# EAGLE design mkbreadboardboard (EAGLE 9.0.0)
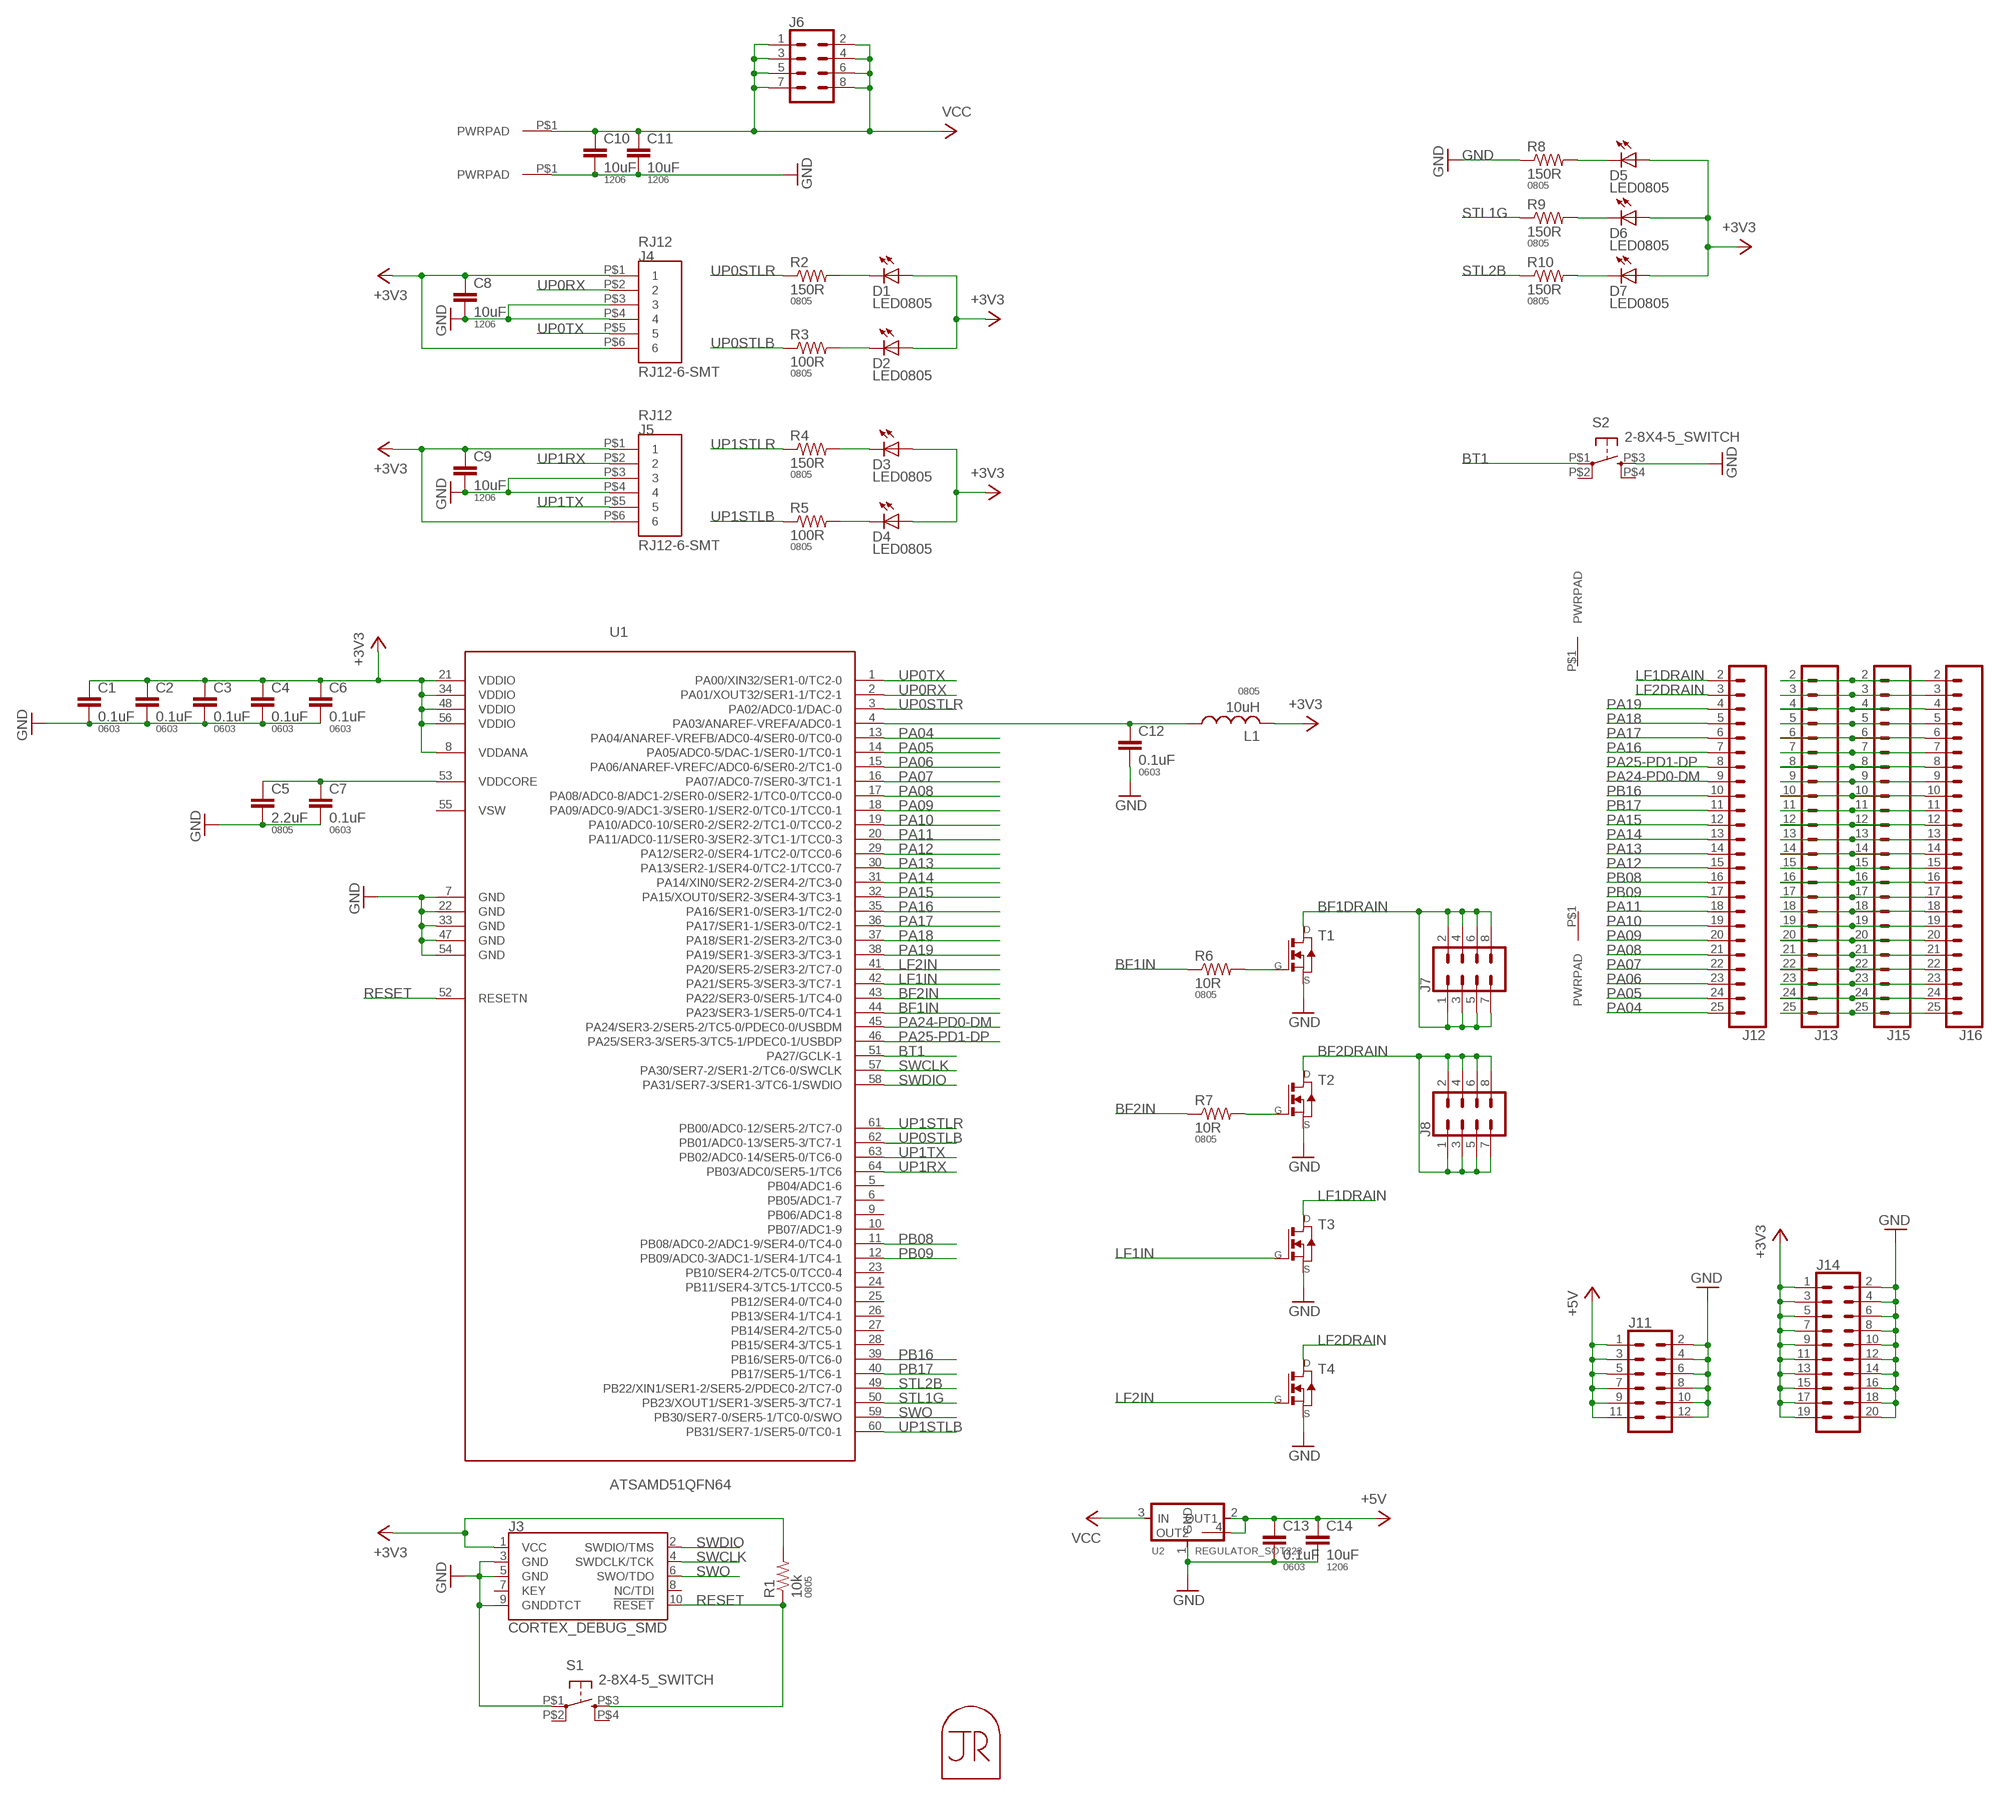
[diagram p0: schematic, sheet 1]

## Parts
C1  0.1uF  CAP0603-CAP  [0603-CAP]
C2  0.1uF  CAP0603-CAP  [0603-CAP]
C3  0.1uF  CAP0603-CAP  [0603-CAP]
C4  0.1uF  CAP0603-CAP  [0603-CAP]
C5  2.2uF  CAP0805  [0805]
C6  0.1uF  CAP0603-CAP  [0603-CAP]
C7  0.1uF  CAP0603-CAP  [0603-CAP]
C8  10uF  CAP1206  [1206]
C9  10uF  CAP1206  [1206]
C10  10uF  CAP1206  [1206]
C11  10uF  CAP1206  [1206]
C12  0.1uF  CAP0603-CAP  [0603-CAP]
C13  0.1uF  CAP0603-CAP  [0603-CAP]
C14  10uF  CAP1206  [1206]
D1  LED0805  [LED0805]
D2  LED0805  [LED0805]
D3  LED0805  [LED0805]
D4  LED0805  [LED0805]
D5  LED0805  [LED0805]
D6  LED0805  [LED0805]
D7  LED0805  [LED0805]
J1  PWRPAD  [PWRPAD_M3-PEM-MOUNT]
J2  PWRPAD  [PWRPAD_M3-PEM-MOUNT]
J3  CORTEX_DEBUG_SMD  [SAMTECH_FTSH-105-01]
J4  RJ12-6-SMT  [RJ12-6-SMT]
J5  RJ12-6-SMT  [RJ12-6-SMT]
J6  CONN_04X2  [2X4]
J7  CONN_04X2  [2X4]
J8  CONN_04X2  [2X4]
J9  PWRPADM3  [PWRPAD_3-25MM]
J10  PWRPADM3  [PWRPAD_3-25MM]
J11  CONN_06X2NO_SILK  [2X6_NOSILK]
J12  CONN_24  [1X24]
J13  CONN_24  [1X24]
J14  CONN_10X2NOSILK  [2X10_NOSILK]
J15  CONN_24  [1X24]
J16  CONN_24  [1X24]
L1  10uH  INDUCTOR-0805  [0805]
MP1  JRTOMBSTONE  [JRTOMBSTONE]
R1  10k  RESISTOR0805-RES  [0805]
R2  150R  RESISTOR0805-RES  [0805]
R3  100R  RESISTOR0805-RES  [0805]
R4  150R  RESISTOR0805-RES  [0805]
R5  100R  RESISTOR0805-RES  [0805]
R6  10R  RESISTOR0805-RES  [0805]
R7  10R  RESISTOR0805-RES  [0805]
R8  150R  RESISTOR0805-RES  [0805]
R9  150R  RESISTOR0805-RES  [0805]
R10  150R  RESISTOR0805-RES  [0805]
S1  2-8X4-5_SWITCH  [TACT-SWITCH-KMR6]
S2  2-8X4-5_SWITCH  [TACT-SWITCH-KMR6]
T1  NMOSFETTO252  [TO252]
T2  NMOSFETTO252  [TO252]
T3  NMOSFETSOT23  [SOT-23]
T4  NMOSFETSOT23  [SOT-23]
U1  ATSAMD51QFN64  [QFN-64-9X9MM]
U2  REGULATOR_SOT223  [SOT223]

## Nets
+3V3: C1.1 C2.1 C3.1 C4.1 C6.1 C8.1 C9.1 D1.1(A) D2.1(A) D3.1(A) D4.1(A) D5.1(A) D6.1(A) D7.1(A) J3.1(VCC) J4.P$1 J4.P$6 J5.P$1 J5.P$6 J14.1 J14.3 J14.5 J14.7 J14.9 J14.11 J14.13 J14.15 J14.17 J14.19 L1.2 R1.2 U1.8(VDDANA) U1.21(VDDIO) U1.34(VDDIO) U1.48(VDDIO) U1.56(VDDIO)
+5V: C13.1 C14.1 J11.1 J11.3 J11.5 J11.7 J11.9 J11.11 U2.2(OUT1) U2.4(OUT2)
BF1DRAIN: J7.1 J7.2 J7.3 J7.4 J7.5 J7.6 J7.7 J7.8 T1.3(D)
BF1IN: R6.1 U1.44(PA23/SER3-1/SER5-0/TC4-1)
BF2DRAIN: J8.1 J8.2 J8.3 J8.4 J8.5 J8.6 J8.7 J8.8 T2.3(D)
BF2IN: R7.1 U1.43(PA22/SER3-0/SER5-1/TC4-0)
BT1: S2.P$1(P) U1.51(PA27/GCLK-1)
GND: C1.2 C2.2 C3.2 C4.2 C5.2 C6.2 C7.2 C8.2 C9.2 C10.2 C11.2 C12.2 C13.2 C14.2 J2.P$1(PWRPAD) J3.3(GND) J3.5(GND) J3.9(GNDDTCT) J4.P$3 J4.P$4 J5.P$3 J5.P$4 J11.2 J11.4 J11.6 J11.8 J11.10 J11.12 J14.2 J14.4 J14.6 J14.8 J14.10 J14.12 J14.14 J14.16 J14.18 J14.20 R8.1 S1.P$1(P) S2.P$3(S) T1.2(S) T2.2(S) T3.2(S) T4.2(S) U1.7(GND) U1.22(GND) U1.33(GND) U1.47(GND) U1.54(GND) U2.1(GND)
LF1DRAIN: J12.2 T3.1(D)
LF1IN: T3.3(G) U1.42(PA21/SER5-3/SER3-3/TC7-1)
LF2DRAIN: J12.3 T4.1(D)
LF2IN: T4.3(G) U1.41(PA20/SER5-2/SER3-2/TC7-0)
N$1: J13.7 J15.7 J16.7
N$2: D1.2(C) R2.2
N$3: J13.8 J15.8 J16.8
N$4: D3.2(C) R4.2
N$5: C5.1 C7.1 U1.53(VDDCORE)
N$6: D2.2(C) R3.2
N$7: D4.2(C) R5.2
N$8: C12.1 L1.1 U1.4(PA03/ANAREF-VREFA/ADC0-1)
N$9: D5.2(C) R8.2
N$10: D6.2(C) R9.2
N$11: D7.2(C) R10.2
N$13: R6.2 T1.1(G)
N$14: R7.2 T2.1(G)
N$15: J13.2 J15.2 J16.2
N$16: J13.3 J15.3 J16.3
N$17: J13.4 J15.4 J16.4
N$18: J13.5 J15.5 J16.5
N$19: J13.6 J15.6 J16.6
N$20: J13.9 J15.9 J16.9
N$21: J13.10 J15.10 J16.10
N$22: J13.11 J15.11 J16.11
N$23: J13.12 J15.12 J16.12
N$24: J13.13 J15.13 J16.13
N$25: J13.14 J15.14 J16.14
N$26: J13.15 J15.15 J16.15
N$27: J13.16 J15.16 J16.16
N$28: J13.17 J15.17 J16.17
N$29: J13.18 J15.18 J16.18
N$30: J13.19 J15.19 J16.19
N$31: J13.20 J15.20 J16.20
N$32: J13.21 J15.21 J16.21
N$33: J13.22 J15.22 J16.22
N$34: J13.23 J15.23 J16.23
N$35: J13.24 J15.24 J16.24
N$36: J13.25 J15.25 J16.25
PA04: J12.25 U1.13(PA04/ANAREF-VREFB/ADC0-4/SER0-0/TC0-0)
PA05: J12.24 U1.14(PA05/ADC0-5/DAC-1/SER0-1/TC0-1)
PA06: J12.23 U1.15(PA06/ANAREF-VREFC/ADC0-6/SER0-2/TC1-0)
PA07: J12.22 U1.16(PA07/ADC0-7/SER0-3/TC1-1)
PA08: J12.21 U1.17(PA08/ADC0-8/ADC1-2/SER0-0/SER2-1/TC0-0/TCC0-0)
PA09: J12.20 U1.18(PA09/ADC0-9/ADC1-3/SER0-1/SER2-0/TC0-1/TCC0-1)
PA10: J12.19 U1.19(PA10/ADC0-10/SER0-2/SER2-2/TC1-0/TCC0-2)
PA11: J12.18 U1.20(PA11/ADC0-11/SER0-3/SER2-3/TC1-1/TCC0-3)
PA12: J12.15 U1.29(PA12/SER2-0/SER4-1/TC2-0/TCC0-6)
PA13: J12.14 U1.30(PA13/SER2-1/SER4-0/TC2-1/TCC0-7)
PA14: J12.13 U1.31(PA14/XIN0/SER2-2/SER4-2/TC3-0)
PA15: J12.12 U1.32(PA15/XOUT0/SER2-3/SER4-3/TC3-1)
PA16: J12.7 U1.35(PA16/SER1-0/SER3-1/TC2-0)
PA17: J12.6 U1.36(PA17/SER1-1/SER3-0/TC2-1)
PA18: J12.5 U1.37(PA18/SER1-2/SER3-2/TC3-0)
PA19: J12.4 U1.38(PA19/SER1-3/SER3-3/TC3-1)
PA24-PD0-DM: J12.9 U1.45(PA24/SER3-2/SER5-2/TC5-0/PDEC0-0/USBDM)
PA25-PD1-DP: J12.8 U1.46(PA25/SER3-3/SER5-3/TC5-1/PDEC0-1/USBDP)
PB08: J12.16 U1.11(PB08/ADC0-2/ADC1-9/SER4-0/TC4-0)
PB09: J12.17 U1.12(PB09/ADC0-3/ADC1-1/SER4-1/TC4-1)
PB16: J12.10 U1.39(PB16/SER5-0/TC6-0)
PB17: J12.11 U1.40(PB17/SER5-1/TC6-1)
RESET: J3.10(!RESET) R1.1 S1.P$3(S) U1.52(RESETN)
STL1G: R9.1 U1.50(PB23/XOUT1/SER1-3/SER5-3/TC7-1)
STL2B: R10.1 U1.49(PB22/XIN1/SER1-2/SER5-2/PDEC0-2/TC7-0)
SWCLK: J3.4(SWDCLK/TCK) U1.57(PA30/SER7-2/SER1-2/TC6-0/SWCLK)
SWDIO: J3.2(SWDIO/TMS) U1.58(PA31/SER7-3/SER1-3/TC6-1/SWDIO)
SWO: J3.6(SWO/TDO) U1.59(PB30/SER7-0/SER5-1/TC0-0/SWO)
UP0RX: J4.P$2 U1.2(PA01/XOUT32/SER1-1/TC2-1)
UP0STLB: R3.1 U1.62(PB01/ADC0-13/SER5-3/TC7-1)
UP0STLR: R2.1 U1.3(PA02/ADC0-1/DAC-0)
UP0TX: J4.P$5 U1.1(PA00/XIN32/SER1-0/TC2-0)
UP1RX: J5.P$2 U1.64(PB03/ADC0/SER5-1/TC6)
UP1STLB: R5.1 U1.60(PB31/SER7-1/SER5-0/TC0-1)
UP1STLR: R4.1 U1.61(PB00/ADC0-12/SER5-2/TC7-0)
UP1TX: J5.P$5 U1.63(PB02/ADC0-14/SER5-0/TC6-0)
VCC: C10.1 C11.1 J1.P$1(PWRPAD) J6.1 J6.2 J6.3 J6.4 J6.5 J6.6 J6.7 J6.8 U2.3(IN)
Unconnected: J3.7(KEY) J3.8(NC/TDI) J9.P$1(PWRPAD) J10.P$1(PWRPAD) S1.P$2(P1) S1.P$4(S1) S2.P$2(P1) S2.P$4(S1) U1.5(PB04/ADC1-6) U1.6(PB05/ADC1-7) U1.9(PB06/ADC1-8) U1.10(PB07/ADC1-9) U1.23(PB10/SER4-2/TC5-0/TCC0-4) U1.24(PB11/SER4-3/TC5-1/TCC0-5) U1.25(PB12/SER4-0/TC4-0) U1.26(PB13/SER4-1/TC4-1) U1.27(PB14/SER4-2/TC5-0) U1.28(PB15/SER4-3/TC5-1) U1.55(VSW)

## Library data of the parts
C1-C4 C6 C7 C12 C13 = borkedlabs-passives:CAP: Capacitor; PACKAGE: 0603
C5 = borkedlabs-passives:CAP: Capacitor; PACKAGE: 0805
C8-C11 C14 = borkedlabs-passives:CAP: Capacitor; PACKAGE: 1206
D1-D7 = lights:LED: LED
J1 J2 J9 J10 = power:PWRPAD
J3 = SparkFun-Connectors:CORTEX_DEBUG: Cortex Debug Connector - 10 pin Supports JTAG debug, Serial Wire debug, and Serial Wire Viewer. PTH and SMD connector options available. General Connector Information Products: PTH Connector -via Digi-Key SparkFun PSoc SparkFun T
J4 J5 = connector:RJ12-6-SMT
J6-J8 = SparkFun-Connectors:CONN_04X2: Multi connection point. Often used as Generic Header-pin footprint for 0.1 inch spaced/style header connections On any of the 0.1 inch spaced packages, you can populate with these: Break Away Headers - Straight (PRT-00116) Break Away Male Headers - Right Angle (PRT-00553) Female Headers (PRT-00115)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
J11 = SparkFun-Connectors:CONN_06X2: Multi connection point. Often used as Generic Header-pin footprint for 0.1 inch spaced/style header connections On any of the 0.1 inch spaced packages, you can populate with these: Break Away Headers - Straight (PRT-00116) Break Away Male Headers - Right Angle (PRT-00553) Female Headers (PRT-00115)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
J12 J13 J15 J16 = SparkFun-Connectors:CONN_24: Multi connection point. Often used as Generic Header-pin footprint for 0.1 inch spaced/style header connections On any of the 0.1 inch spaced packages, you can populate with these: Break Away Headers - Straight (PRT-00116) Break Away Male Headers - Right Angle (PRT-00553) Female Headers (PRT-00115)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
J14 = SparkFun-Connectors:CONN_10X2: Multi connection point. Often used as Generic Header-pin footprint for 0.1 inch spaced/style header connections On any of the 0.1 inch spaced packages, you can populate with these: Break Away Headers - Straight (PRT-00116) Break Away Male Headers - Right Angle (PRT-00553) Female Headers (PRT-00115)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
L1 = borkedlabs-passives:INDUCTOR; PACKAGE: 0805
MP1 = connector:JRTOMBSTONE
R1-R10 = borkedlabs-passives:RESISTOR: Resistor; PACKAGE: 0805
S1 S2 = fab:2-8X4-5_SWITCH
T1-T4 = fab:NMOSFET: MOS FET
U1 = microcontrollers:ATSAMD51
U2 = fab:REGULATOR_SOT223

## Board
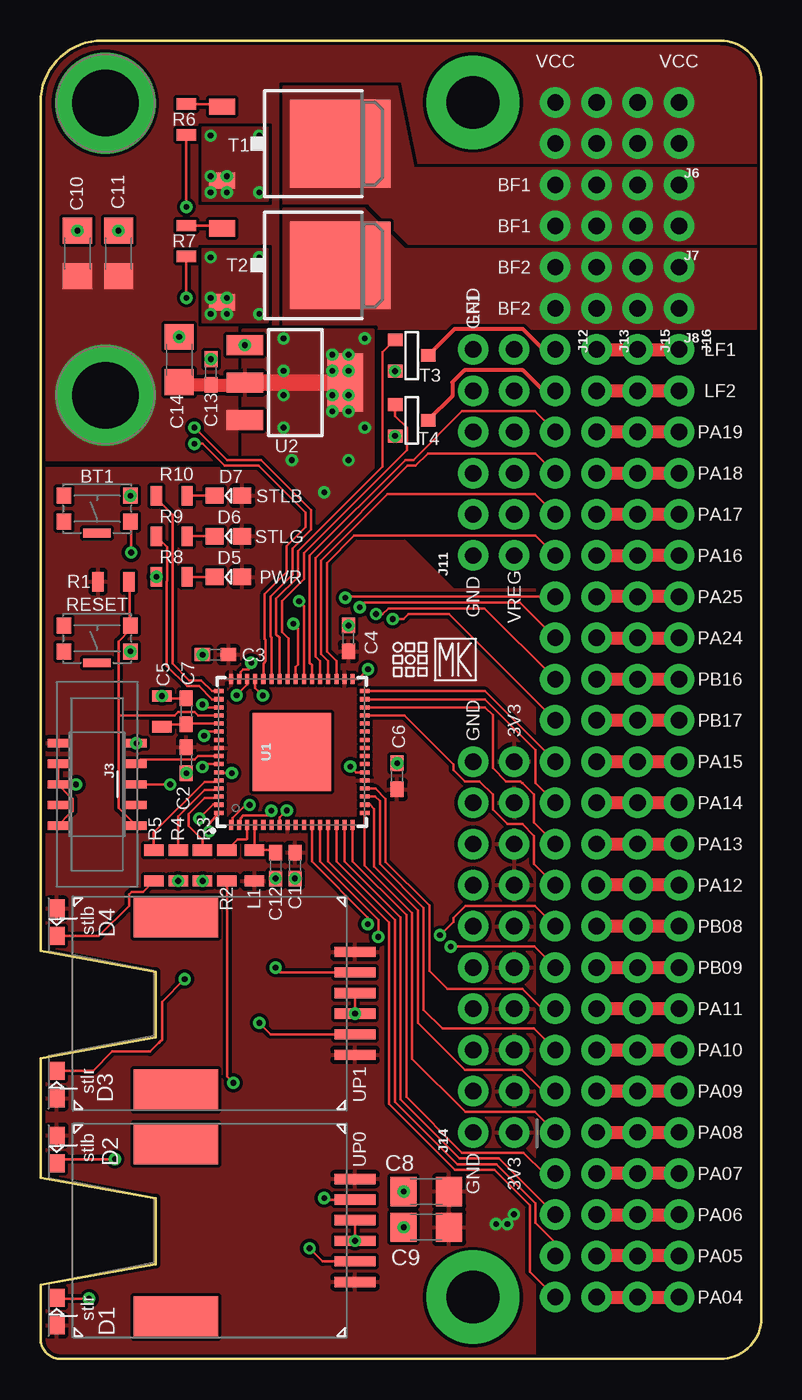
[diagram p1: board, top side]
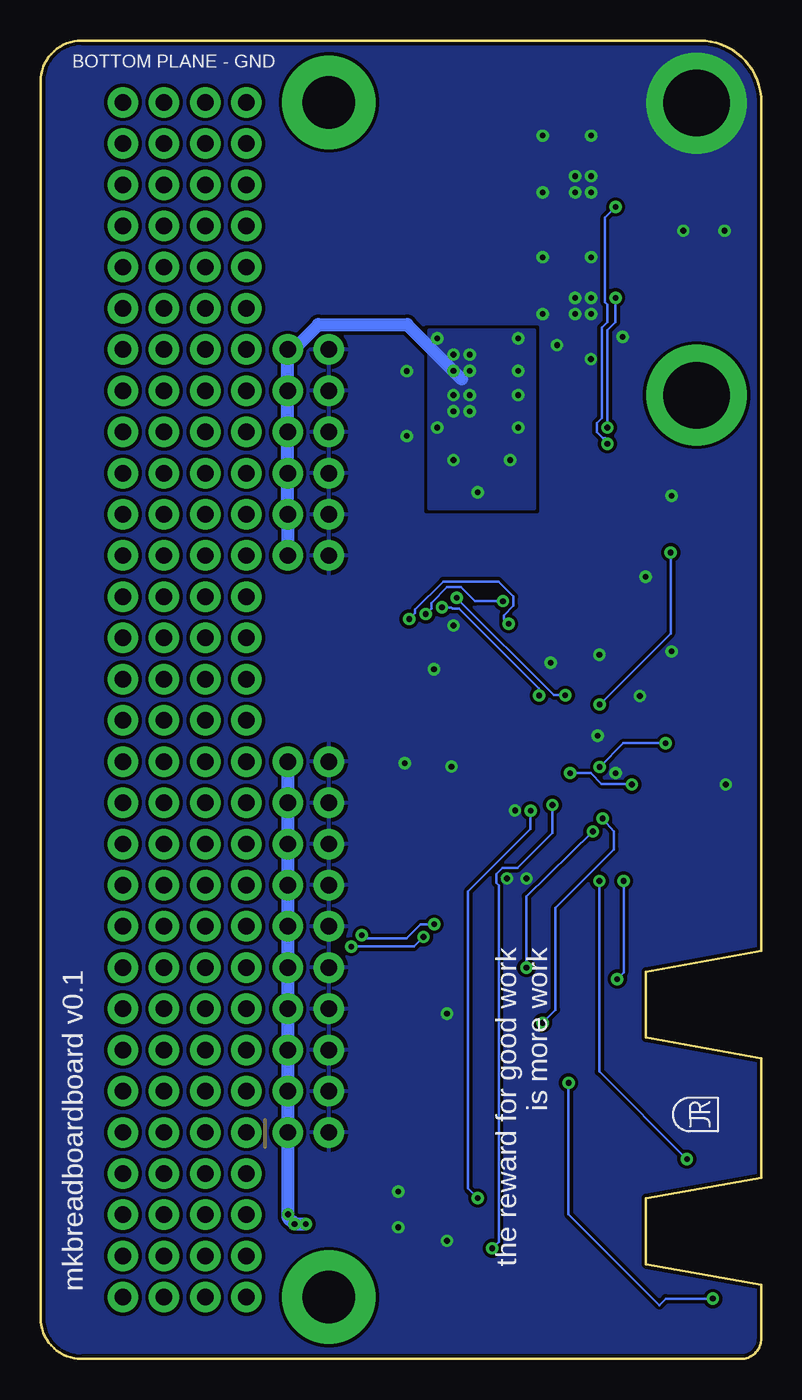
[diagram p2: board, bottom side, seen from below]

Size 44.45 x 81.28 mm. Coordinates in mm from the lower left corner, seen from the top.
Outline: 41.91,81.28 3.81,81.28 arc90 0,77.47 0,25.15 7.11,23.88 7.11,19.81 0,18.54 0,11.18 7.11,9.91 7.11,5.84 0,4.57 0,1.27 arc90 1.27,0 41.91,0 arc90 44.45,2.54 44.45,78.74 arc90 41.91,81.28
Copper layers (1*16): Top 0.035mm / dielectric 1.5mm / Bottom 0.035mm
Design rules "default *": minimum track width 6mil, minimum drill 0.35mm, track to track 8mil, track to pad 8mil, pad to pad 8mil, via to via 8mil, smd to smd 8mil, copper to edge 8mil, drill to drill 8mil, minimum pad ring 10mil, minimum via ring 8mil, stop-mask expansion 4mil, vias tented up to drill 25mil, thermal gap 10mil

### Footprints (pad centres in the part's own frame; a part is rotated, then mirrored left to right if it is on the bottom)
0603-CAP = smd 0.96 x 0.8: 1 -0.8,0; 2 0.8,0
0805 = smd 0.7 x 1.2: 1 -0.95,0; 2 0.95,0
1206 = smd 1.6 x 1.8: 1 -1.4,0; 2 1.4,0
LED0805 = smd 1.1 x 1: 1 -0.85,0; 2 0.85,0
PWRPAD_M3-PEM-MOUNT = drill 4.1 pad 6.2: P$1 0,0
SAMTECH_FTSH-105-01 = smd 0.508 x 1.27: 1 -2.54,-2.413; 2 -2.54,2.413; 3 -1.27,-2.413; 4 -1.27,2.413; 5 0,-2.413; 6 0,2.413; 7 1.27,-2.413; 8 1.27,2.413; 9 2.54,-2.413; 10 2.54,2.413
RJ12-6-SMT = smd 0.635 x 2.54: P$1 -3.175,17.399; P$2 -1.905,17.399; P$3 -0.635,17.399; P$4 0.635,17.399; P$5 1.905,17.399; P$6 3.175,17.399 | smd 2.54 x 5.207: P$7 -5.334,6.35; P$8 5.334,6.35
2X4 = drill 1.016 pad 1.88: 1 -3.81,-1.27; 2 -3.81,1.27; 3 -1.27,-1.27; 4 -1.27,1.27; 5 1.27,-1.27; 6 1.27,1.27; 7 3.81,-1.27; 8 3.81,1.27
PWRPAD_3-25MM = drill 3.25 pad 5.75: P$1 0,0
2X6_NOSILK = drill 1.016 pad 1.88: 1 0,0; 2 0,2.54; 3 2.54,0; 4 2.54,2.54; 5 5.08,0; 6 5.08,2.54; 7 7.62,0; 8 7.62,2.54; 9 10.16,0; 10 10.16,2.54; 11 12.7,0; 12 12.7,2.54
1X24 = drill 1.016 pad 1.88: 2 -26.67,0; 3 -24.13,0; 4 -21.59,0; 5 -19.05,0; 6 -16.51,0; 7 -13.97,0; 8 -11.43,0; 9 -8.89,0; 10 -6.35,0; 11 -3.81,0; 12 -1.27,0; 13 1.27,0; 14 3.81,0; 15 6.35,0; 16 8.89,0; 17 11.43,0; 18 13.97,0; 19 16.51,0; 20 19.05,0; 21 21.59,0; 22 24.13,0; 23 26.67,0; 24 29.21,0; 25 31.75,0
2X10_NOSILK = drill 1.016 pad 1.88: 1 0,0; 2 0,2.54; 3 2.54,0; 4 2.54,2.54; 5 5.08,0; 6 5.08,2.54; 7 7.62,0; 8 7.62,2.54; 9 10.16,0; 10 10.16,2.54; 11 12.7,0; 12 12.7,2.54; 13 15.24,0; 14 15.24,2.54; 15 17.78,0; 16 17.78,2.54; 17 20.32,0; 18 20.32,2.54; 19 22.86,0; 20 22.86,2.54
TACT-SWITCH-KMR6 = smd 0.9 x 1: P$1 -2.05,0.8; P$2 2.05,0.8; P$3 -2.05,-0.8; P$4 2.05,-0.8 | smd 1.7 x 0.55: P$5 0,1.5
TO252 = smd 1 x 1.6: 1 -2.28,-4.8; 2 2.28,-4.8 | smd 5.4 x 6.2: 3 0,2.5
SOT-23 = smd 0.787 x 0.889: 1 0.025,-1.016; 2 -0.94,1.016; 3 0.991,1.016
QFN-64-9X9MM = smd 0.6 x 0.25: 1 -4.5,3.75; 2 -4.5,3.25; 3 -4.5,2.75; 4 -4.5,2.25; 5 -4.5,1.75; 6 -4.5,1.25; 7 -4.5,0.75; 8 -4.5,0.25; 9 -4.5,-0.25; 10 -4.5,-0.75; 11 -4.5,-1.25; 12 -4.5,-1.75; 13 -4.5,-2.25; 14 -4.5,-2.75; 15 -4.5,-3.25; 16 -4.5,-3.75; 33 4.5,-3.75; 34 4.5,-3.25; 35 4.5,-2.75; 36 4.5,-2.25; 37 4.5,-1.75; 38 4.5,-1.25; 39 4.5,-0.75; 40 4.5,-0.25; 41 4.5,0.25; 42 4.5,0.75; 43 4.5,1.25; 44 4.5,1.75; 45 4.5,2.25; 46 4.5,2.75; 47 4.5,3.25; 48 4.5,3.75 | smd 0.25 x 0.6: 17 -3.75,-4.5; 18 -3.25,-4.5; 19 -2.75,-4.5; 20 -2.25,-4.5; 21 -1.75,-4.5; 22 -1.25,-4.5; 23 -0.75,-4.5; 24 -0.25,-4.5; 25 0.25,-4.5; 26 0.75,-4.5; 27 1.25,-4.5; 28 1.75,-4.5; 29 2.25,-4.5; 30 2.75,-4.5; 31 3.25,-4.5; 32 3.75,-4.5; 49 3.75,4.5; 50 3.25,4.5; 51 2.75,4.5; 52 2.25,4.5; 53 1.75,4.5; 54 1.25,4.5; 55 0.75,4.5; 56 0.25,4.5; 57 -0.25,4.5; 58 -0.75,4.5; 59 -1.25,4.5; 60 -1.75,4.5; 61 -2.25,4.5; 62 -2.75,4.5; 63 -3.25,4.5; 64 -3.75,4.5 | smd 4.826 x 4.826: P$1 0,0
SOT223 = smd 1.219 x 2.235: 1 -2.311,-3.099; 2 0,-3.099; 3 2.311,-3.099 | smd 3.6 x 2.2: 4 0,3.099

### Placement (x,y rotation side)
C1  15.69,30.42 270 top
C2  8.99,36.92 270 top
C3  10.79,43.42 180 top
C4  18.99,44.42 90 top
C5  7.49,39.92 90 top
C6  21.99,35.92 90 top
C7  8.99,39.92 90 top
C8  23.79,10.32 180 top
C9  23.79,8.12 180 top
C10  2.27,68.16 90 top
C11  4.81,68.16 90 top
C12  14.49,30.42 270 top
C13  10.51,60.84 90 top
C14  8.55,61.61 90 top
D1  0.99,2.92 90 top
D2  0.99,12.92 270 top
D3  0.99,16.92 90 top
D4  0.99,26.92 270 top
D5  11.59,48.22 180 top
D6  11.59,50.72 180 top
D7  11.59,53.22 180 top
J1  3.99,59.42 0 top
J2  3.99,77.42 0 top
J3  3.49,35.42 270 top
J4  1.99,7.92 270 top
J5  1.99,21.92 270 top
J6  35.56,76.2 180 top
J7  35.56,71.12 180 top
J8  35.56,66.04 180 top
J9  26.67,77.47 0 top
J10  26.67,3.81 0 top
J11  29.21,49.53 90 top
J12  31.75,35.56 270 top
J13  34.29,35.56 270 top
J14  29.21,13.97 90 top
J15  36.83,35.56 270 top
J16  39.37,35.56 270 top
L1  13.19,30.42 270 top
MP1  3.69,15.12 90 bottom
R1  4.49,47.92 180 top
R2  11.49,30.42 270 top
R3  9.99,30.42 270 top
R4  8.49,30.42 270 top
R5  6.99,30.42 270 top
R6  8.99,76.42 90 top
R7  8.99,68.92 90 top
R8  8.09,48.22 0 top
R9  8.09,50.72 0 top
R10  8.09,53.22 0 top
S1  3.49,44.42 180 top
S2  3.49,52.42 180 top
T1  15.99,74.92 270 top
T2  15.99,67.42 270 top
T3  22.88,61.84 90 top
T4  22.88,57.84 90 top
U1  15.49,37.42 90 top
U2  15.7,60.19 270 top
U$6  CBA-LOGO  [CBA-SILK-LOGO]  22.79,43.12 0 top
U$10  MK-LOGO  [MK-LOGO-SILK]  25.59,43.12 0 top

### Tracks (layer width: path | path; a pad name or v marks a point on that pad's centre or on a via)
+3V3  (via drill 0.35)
  Bottom 0.813: J14.19 J14.17 J14.15 J14.13 J14.11 J14.9 J14.7 J14.5 J14.3 J14.1 29.21,8.74 v28.79,8.32 v28.09,8.32
  other vias: 29.19,8.92
  pour Top (rank 2): -1.01,-0.58 -1.01,54.92 17.99,54.92 25.49,47.42 30.49,47.42 30.49,-0.58
+5V  (via drill 0.35)
  Top 0.813: U2.2 12.45,60.04 C13.1 8.72,60.04 C14.1
  Top 1.016: U2.2 U2.4
  Bottom 0.813: 18.49,60.42 21.85,63.78 27.31,63.78 28.86,62.23 J11.11 J11.9 J11.7 J11.5 J11.3 J11.1
  other vias: 19.99,62.92 14.99,62.92 14.99,57.42 19.99,57.42 18.99,58.42 17.99,58.42 17.99,59.42 18.99,59.42 18.99,60.92 17.99,60.92 17.99,61.92 18.99,61.92 14.99,59.42 14.99,60.92 15.49,55.42 17.49,53.42 18.99,55.42
  pour Top: 12.49,63.42 12.49,55.42 13.49,55.42 16.49,52.42 16.49,50.92 20.49,51.92 20.49,63.42
  pour Bottom: 20.49,63.42 13.99,63.42 13.99,52.42 20.49,52.42
BF1DRAIN
  pour Top (rank 3, no thermals): 14.99,70.92 19.99,70.92 22.49,68.42 44.49,68.42 44.49,73.42 22.99,73.42 21.99,78.42 14.99,78.42
BF1IN  (via drill 0.35)
  Top 0.152: U1.44 13.74,42.87 13.88,43.01 13.88,44.32 13.82,44.38 13.82,47.16 15.17,48.51 15.17,50.11 16.33,51.27 16.33,52.17 13.44,55.06 11.34,55.06 9.99,56.42 v9.49,56.42 | v8.99,71.02 R6.1
  Bottom 0.152: v9.49,56.42 9.39,56.52 9.63,56.76 9.76,56.76 10.15,57.15 10.15,57.69 9.85,57.99 9.85,63.57 9.49,63.92 9.49,64.99 9.65,65.15 9.65,70.36 v8.99,71.02
BF2DRAIN
  pour Top (rank 2, no thermals): 44.49,68.42 22.49,68.42 19.99,70.92 14.99,70.92 14.99,63.52 44.49,63.52
BF2IN  (via drill 0.35)
  Top 0.152: R7.1 v8.99,65.42 | v9.49,57.42 11.49,55.42 13.59,55.42 16.69,52.32 16.69,51.13 15.53,49.97 15.53,48.37 14.18,47.02 14.18,44.52 14.24,44.46 U1.43
  Bottom 0.152: v8.99,65.42 8.99,63.92 9.49,63.42 v9.49,57.42
BT1  (via drill 0.35)
  Top 0.152: S2.P$1 5.59,51.57 v5.59,49.72 | v9.97,40.34 10.14,40.17 U1.51
  Bottom 0.152: v5.59,49.72 5.59,44.73 v9.97,40.34
GND  (via drill 0.35)
  Top 0.152: v12.99,42.92 12.99,42.67 12.82,42.5 12.5,42.5 12.34,42.34 12.34,42.02 U1.47 | J3.3 J3.5 | J3.5 1.81,34.68 1.83,34.68 1.99,34.52 1.99,33.78 1.83,33.62 1.81,33.62 J3.9 | J3.5 v2.19,35.42 | C7.2 7.64,40.72 C5.2 | U1.54 10.34,38.67 v10.09,38.42 | U1.22 19.46,36.17 v19.11,36.52 | U1.7 14.74,33.37 v15.19,33.82 | U1.33 19.59,41.92 v20.19,42.52 | J5.P$3 J5.P$4 | J4.P$3 v19.39,7.28
  other vias: 21.86,56.9 21.86,60.9 9.99,43.42 5.54,43.62 7.49,40.87 8.99,36.12 18.99,45.22 21.99,36.72 15.69,29.62 14.49,29.62 22.39,10.32 22.39,8.12 12.6,62.5 10.51,61.64 8.55,63.01 10.49,64.42 11.49,64.42 11.49,65.42 10.49,65.42 10.49,67.92 13.49,67.92 13.49,64.42 10.49,71.92 11.49,71.92 11.49,72.92 10.49,72.92 10.49,75.42 13.49,75.42 13.49,71.92 4.81,69.56 2.27,69.56 5.54,53.22 7.14,48.22 19.39,21.29
  pour Bottom (rank 6): -0.51,81.92 46.3,81.92 46.3,-0.58 -0.51,-0.58
  pour Top (no thermals): 13.99,63.92 9.99,63.92 9.99,68.42 13.99,68.42
  pour Top (no thermals): 13.99,71.42 9.99,71.42 9.99,75.92 13.99,75.92
LF1DRAIN
  Top 0.254: J12.2 31.01,62.23 29.74,63.5 25.53,63.5 T3.1
LF1IN
  Top 0.152: U1.42 14.74,44.47 14.53,44.67 14.53,46.87 15.88,48.22 15.88,49.82 21.09,55.02 21.09,62.06 T3.3
LF2DRAIN
  Top 0.254: J12.3 31.01,59.69 29.74,60.96 26.14,60.96 25.4,60.22 25.4,59.37 T4.1
LF2IN
  Top 0.152: T4.3 21.86,58.13 22.59,57.41 22.59,56.02 16.24,49.67 16.24,48.07 14.89,46.72 14.89,44.82 15.29,44.42 15.29,41.97 U1.41
N$1
  Top 0.813: J13.7 J15.7 J16.7
N$2  (via drill 0.35)
  Top 0.152: R2.2 11.49,17.42 v11.89,17.02 | v2.99,3.72 1.04,3.72 D1.2
  Bottom 0.152: v11.89,17.02 11.89,8.92 6.29,3.32 5.89,3.72 v2.99,3.72
N$3
  Top 0.813: J13.8 J15.8 J16.8
N$4  (via drill 0.35)
  Top 0.152: D3.2 3.24,17.77 4.42,18.95 6.75,18.95 7.28,19.48 7.32,19.49 7.39,19.58 7.49,19.69 7.49,22.02 v8.89,23.42
  Bottom 0.152: R4.2 8.49,23.82 v8.89,23.42
  other vias: 8.49,29.47
N$5
  Top 0.152: U1.53 9.04,39.17 C7.1 7.64,39.12 C5.1
N$6  (via drill 0.35)
  Top 0.152: v4.59,12.32 0.69,12.32 | 0.69,12.32 0.59,12.42 | 0.69,12.32 0.94,12.07 D2.2
  Bottom 0.152: R3.2 9.99,17.72 v4.59,12.32
  other vias: 9.99,29.47
N$7
  Top 0.152: D4.2 3.59,26.07 5.46,27.94 5.46,28.64 5.62,28.8 6.32,28.8 R5.2
N$8
  Top 0.152: C12.1 14.34,31.37 L1.1 13.19,32.87 U1.4
N$9
  Top 0.152: R8.2 D5.2
N$10
  Top 0.152: R9.2 D6.2
N$11
  Top 0.152: R10.2 D7.2
N$13
  Top 0.152: R6.2 11.02,77.37 T1.1
N$14
  Top 0.152: R7.2 11.02,69.87 T2.1
N$15
  Top 0.813: J13.2 J15.2 J16.2
N$16
  Top 0.813: J13.3 J15.3 J16.3
N$17
  Top 0.813: J16.4 J15.4 J13.4
N$18
  Top 0.813: J13.5 J15.5 J16.5
N$19
  Top 0.813: J16.6 J15.6 J13.6
N$20
  Top 0.813: J13.9 J15.9 J16.9
N$21
  Top 0.813: J13.10 J15.10 J16.10
N$22
  Top 0.813: J16.11 J15.11 J13.11
N$23
  Top 0.813: J13.12 J15.12 J16.12
N$24
  Top 0.813: J16.13 J15.13 J13.13
N$25
  Top 0.813: J13.14 J15.14 J16.14
N$26
  Top 0.813: J16.15 J15.15 J13.15
N$27
  Top 0.813: J16.16 J15.16 J13.16
N$28
  Top 0.813: J13.17 J15.17 J16.17
N$29
  Top 0.813: J16.18 J15.18 J13.18
N$30
  Top 0.813: J13.19 J15.19 J16.19
N$31
  Top 0.813: J16.20 J15.20 J13.20
N$32
  Top 0.813: J13.21 J15.21 J16.21
N$33
  Top 0.813: J16.22 J15.22 J13.22
N$34
  Top 0.813: J13.23 J15.23 J16.23
N$35
  Top 0.813: J16.24 J15.24 J13.24
N$36
  Top 0.813: J13.25 J15.25 J16.25
PA04
  Top 0.152: U1.13 17.74,30.67 21.49,26.92 21.49,15.71 25.55,11.65 27.98,11.65 30.18,9.46 30.18,5.38 J12.25
PA05
  Top 0.152: U1.14 18.24,30.67 21.85,27.07 21.85,15.86 25.7,12.01 28.13,12.01 30.53,9.61 30.53,8.39 31.75,7.17 J12.24
PA06
  Top 0.152: U1.15 18.74,30.68 22.2,27.21 22.2,16.01 25.84,12.36 28.28,12.36 J12.23
PA07
  Top 0.152: U1.16 19.24,30.68 22.56,27.36 22.56,16.15 25.99,12.72 29.79,12.72 31.08,11.43 J12.22
PA08
  Top 0.152: U1.17 19.99,30.43 22.91,27.51 22.91,18.5 26.19,15.22 30.5,15.22 J12.21
PA09
  Top 0.152: U1.18 20.31,34.17 20.57,33.91 20.57,30.36 23.27,27.66 23.27,20.73 26.17,17.83 29.68,17.83 31,16.51 J12.20
PA10
  Top 0.152: U1.19 20.64,34.67 20.93,34.38 20.93,30.5 23.62,27.8 23.62,21.52 24.77,20.37 30.43,20.37 J12.19
PA11
  Top 0.152: J12.18 30.93,21.59 29.71,22.81 25.1,22.81 23.98,23.93 23.98,27.95 21.28,30.65 21.28,34.53 20.64,35.17 U1.20
PA12
  Top 0.152: J12.15 30.43,30.53 30.43,32.26 29.71,32.97 28.81,32.97 27.89,33.89 27.89,34.8 27.07,35.61 26.17,35.61 25.45,36.33 25.45,36.65 22.43,39.67 U1.29
PA13
  Top 0.152: J12.14 30.43,33.07 30.43,34.8 29.71,35.51 29.7,35.51 29.6,35.61 28.71,35.61 27.89,36.43 27.89,39.69 27.4,40.17 U1.30
PA14
  Top 0.152: J12.13 30.53,35.51 30.53,37.55 27.41,40.67 U1.31
PA15
  Top 0.152: J12.12 27.41,41.17 U1.32
PA16
  Top 0.152: U1.35 18.24,43.04 17.66,43.62 17.66,49.08 19.33,50.75 30.53,50.75 J12.7
PA17
  Top 0.152: J12.6 30.5,53.32 21.4,53.32 17.31,49.23 17.31,43.47 17.74,43.03 U1.36
PA18
  Top 0.152: J12.5 30.53,55.83 23.9,55.83 23.14,55.06 22.64,55.06 16.95,49.38 16.95,43.32 17.24,43.03 U1.37
PA19
  Top 0.152: J12.4 30.48,58.42 25.99,58.42 22.99,55.42 22.49,55.42 16.6,49.52 16.6,42.92 16.74,42.78 U1.38
PA24-PD0-DM  (via drill 0.35)
  Top 0.152: J12.9 29.57,46.63 19.99,46.63 v19.69,46.33 | U1.45 13.24,41.37 v13.71,40.91
  Bottom 0.152: v19.69,46.33 19.13,46.33 19.06,46.26 18.64,46.26 13.71,41.33 v13.71,40.91
PA25-PD1-DP  (via drill 0.35)
  Top 0.152: J12.8 18.86,46.99 v18.79,46.92 | v12.09,40.92 12.74,41.57 U1.46
  Bottom 0.152: v18.79,46.92 12.79,40.92 v12.09,40.92
PB08  (via drill 0.35)
  Top 0.152: U1.11 16.74,30.66 20.17,27.23 v20.17,26.8 | v24.64,26.12 25.45,26.94 25.45,27.18 26.2,27.92 30.5,27.92 J12.16
  Bottom 0.152: v20.17,26.8 21.01,26.8 21.89,25.92 24.43,25.92 v24.64,26.12
PB09  (via drill 0.35)
  Top 0.152: J12.17 30.46,25.42 v25.29,25.42 | v20.83,26.02 20.83,27.07 17.24,30.67 U1.12
  Bottom 0.152: v25.29,25.42 21.43,25.42 v20.83,26.02
PB16  (via drill 0.35)
  Top 0.152: U1.39 16.24,46.42 v15.94,46.72 | v20.69,45.92 21.09,45.92 21.45,46.28 27.38,46.28 J12.10
  Bottom 0.152: v20.69,45.92 20.35,46.26 20.35,46.61 19.38,47.58 18.52,47.58 17.66,46.72 v15.94,46.72
PB17  (via drill 0.35)
  Top 0.152: U1.40 15.74,42.67 15.88,42.81 15.88,45.02 v15.58,45.32 | v21.72,45.62 22.39,45.62 22.69,45.92 25.2,45.92 J12.11
  Bottom 0.152: v15.58,45.32 15.88,45.62 15.88,45.84 15.28,46.45 15.28,46.99 16.22,47.93 19.61,47.93 21.35,46.19 21.35,45.99 v21.72,45.62
RESET
  Top 0.152: 4.81,39.72 4.81,33.96 5.15,33.62 5.17,33.62 J3.10 | 4.81,39.72 4.81,44.24 5.54,44.97 S1.P$3 5.49,45.27 5.49,47.37 R1.1 | 4.81,39.72 4.86,39.67 8.26,39.67 8.47,39.88 9.51,39.88 9.71,39.67 U1.52
STL1G
  Top 0.152: U1.50 10.57,40.67 9.77,41.48 9.03,41.48 7.79,42.72 7.79,47.94 7.8,47.95 7.8,50.06 R9.1
STL2B
  Top 0.152: R10.1 7.14,53.07 8.15,52.06 8.15,42.86 9.18,41.84 9.91,41.84 10.58,41.17 U1.49
SWCLK
  Top 0.152: U1.57 9.71,37.17 9.51,36.96 6.17,36.96 J3.4
SWDIO  (via drill 0.35)
  Top 0.152: U1.58 10.14,36.67 v9.97,36.5
  Bottom 0.152: v9.97,36.5 8.51,37.96 J3.2
  other vias: 5.9,37.96
SWO  (via drill 0.35)
  Top 0.152: U1.59 11.04,36.12 v11.79,36.12 | v7.99,35.42 J3.6
  Bottom 0.152: v11.79,36.12 10.53,36.12 9.87,35.46 8.03,35.46 v7.99,35.42
UP0RX  (via drill 0.35)
  Top 0.152: U1.2 12.34,33.02 12.34,33.34 12.5,33.5 14.09,33.5 14.09,33.66 v14.23,33.8 | v17.49,9.92 17.59,9.82 J4.P$2
  Bottom 0.152: v14.23,33.8 14.23,32.68 18.09,28.82 18.09,10.52 v17.49,9.92
UP0STLB
  Top 0.152: U1.62 10.89,34.57 10.11,34.57 9.13,33.59 9.13,32.85 9.99,31.99 R3.1
UP0STLR
  Top 0.152: R2.1 12.14,32.02 12.69,32.02 12.74,32.07 U1.3
UP0TX  (via drill 0.35)
  Top 0.152: J4.P$5 17.39,6.01 v16.59,6.82 | U1.1 11.84,33.02 11.84,33.34 12.65,34.16 v12.89,34.16
  Bottom 0.152: v16.59,6.82 16.19,7.22 16.19,29.19 16.35,29.35 16.35,29.89 15.96,30.28 15.03,30.28 12.89,32.42 v12.89,34.16
UP1RX  (via drill 0.35)
  Top 0.152: U1.64 10.39,32.97 v10.39,32.52 | v14.49,24.12 14.78,23.82 J5.P$2
  Bottom 0.152: v10.39,32.52 14.49,28.52 v14.49,24.12
UP1STLB
  Top 0.152: U1.60 10.89,35.57 10.11,35.57 6.99,32.46 R5.1
UP1STLR
  Top 0.152: U1.61 10.89,35.07 10.11,35.07 8.49,33.45 R4.1
UP1TX  (via drill 0.35)
  Top 0.152: J5.P$5 14.19,20.02 v13.49,20.72 | v9.79,33.32 10.64,34.17 U1.63
  Bottom 0.152: v13.49,20.72 12.69,21.52 12.69,27.82 9.09,31.42 9.09,32.52 v9.79,33.32
VCC
  pour Top (rank 6, no thermals): -1.01,55.42 13.99,55.42 13.99,63.32 48.07,63.32 48.07,82.42 -1.01,82.42

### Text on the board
tPlace: VCC | VCC | BF1 | BF1 | BF2 | GND | LF1 | BF2 | LF1 | LF2 | PA19 | BT1 | PA18 | STLB | PA17 | STLG | PA16 | PWR | GND | VREG | PA25 | RESET | PA24 | PB16 | GND | 3V3 | PB17 | PA15 | PA14 | PA13 | PA12 | PB08 | PB09 | PA11 | PA10 | UP1 | PA09 | PA08 | UP0 | GND | 3V3 | PA07 | PA06 | PA05 | PA04
bPlace: BOTTOM PLANE - GND | the reward for good work / is more work | mkbreadboardboard v0.1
